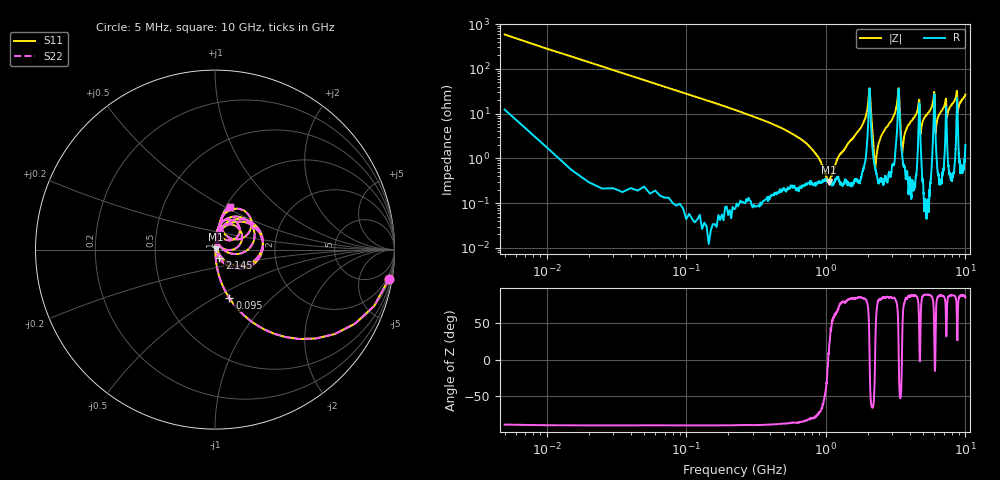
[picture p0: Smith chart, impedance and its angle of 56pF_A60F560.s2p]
! Amotech Co.,Ltd.
! http://www.amotech.co.kr/
! Part Number: A60F560
! These Parameters are Measured in Series Mode Connection
! Operation Temp=25[degC], DC Bias Voltage=0[V]
! Freq. Start=5[MHz] Stop=10[GHz], 2000[Steps]
! Date: Monday, July 20, 2020, 03:42:11
# GHZ S RI R 50.000000
!Freq.(Hz) S11(Real) S11(Imag) S21(Real) S21(Imag) S12(Real) S12(Imag) S22(Real) S22(Imag)
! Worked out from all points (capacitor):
!   2000 points, 5 MHz to 10 GHz, reference 50 ohm
!   read as one part in series: C = 56.4 pF near 55 MHz
!   lowest |Z| = 297 mohm at 1.055 GHz (marker M1)
!   series resonance near 1.04 GHz, so ESL is about 410 pH
!   S11 on the Smith chart (normalised r, x): 5 MHz: 1, -12; 95 MHz: 1.00, -0.59; 2.145 GHz: 1.04, -0.10; 10 GHz: 1.04, +0.53
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0.005  0.9683 -0.1651  0.0317 0.1651  0.0317 0.1651  0.9683 -0.1651
0.095  0.0803 -0.2705  0.9197 0.2705  0.9197 0.2705  0.0803 -0.2705
1.055  0.00286 0.000765  0.9971 -0.000765  0.9971 -0.000765  0.00286 0.000765
1.675  0.00473 0.0372  0.9953 -0.0372  0.9953 -0.0372  0.00473 0.0372
2.045  0.2238 0.1233  0.7762 -0.1233  0.7762 -0.1233  0.2238 0.1233
2.145  0.0239 -0.0463  0.9761 0.0463  0.9761 0.0463  0.0239 -0.0463
2.27  0.00573 0.00362  0.9943 -0.00362  0.9943 -0.00362  0.00573 0.00362
2.5  0.00456 0.0319  0.9954 -0.0319  0.9954 -0.0319  0.00456 0.0319
3.34  0.2421 -0.0374  0.7579 0.0374  0.7579 0.0374  0.2421 -0.0374
3.53  0.0112 0.00686  0.9888 -0.00686  0.9888 -0.00686  0.0112 0.00686
3.76  0.00544 0.0428  0.9946 -0.0428  0.9946 -0.0428  0.00544 0.0428
4.635  0.0875 0.1405  0.9125 -0.1405  0.9125 -0.1405  0.0875 0.1405
4.78  0.0213 0.027  0.9787 -0.027  0.9787 -0.027  0.0213 0.027
5.005  0.00747 0.0734  0.9925 -0.0734  0.9925 -0.0734  0.00747 0.0734
5.955  0.1693 0.1697  0.8307 -0.1697  0.8307 -0.1697  0.1693 0.1697
6.13  0.0249 0.0267  0.9751 -0.0267  0.9751 -0.0267  0.0249 0.0267
6.67  0.0151 0.1079  0.9849 -0.1079  0.9849 -0.1079  0.0151 0.1079
7.375  0.0341 0.0716  0.9659 -0.0716  0.9659 -0.0716  0.0341 0.0716
8.335  0.0419 0.185  0.9581 -0.185  0.9581 -0.185  0.0419 0.185
8.67  0.165 0.2146  0.835 -0.2146  0.835 -0.2146  0.165 0.2146
8.83  0.0524 0.0892  0.9476 -0.0892  0.9476 -0.0892  0.0524 0.0892
10  0.0819 0.2392  0.9181 -0.2392  0.9181 -0.2392  0.0819 0.2392
